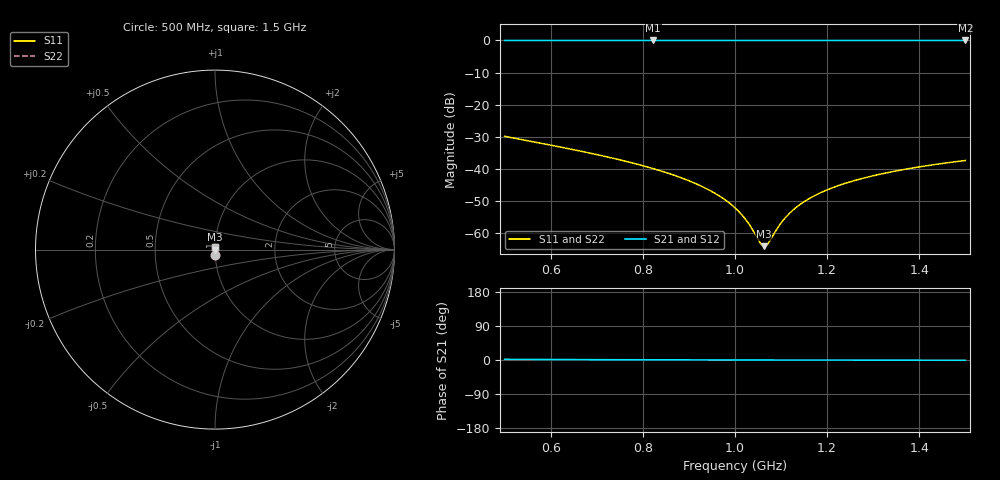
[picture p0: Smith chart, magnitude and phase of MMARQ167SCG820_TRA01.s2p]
! MMARQ167SCG820_TRA01  S-PARAMETER MODEL  ( General Type )
! Model Generated by TAIYO YUDEN Corporation (http://www.ty-top.com)
! Version 1.0
! TAIYO YUDEN Control No. 150609
! Copyright(c) 2015 TAIYO YUDEN CO.,LTD. All Rights Reserved.
! Product Description (link to TY-COMPAS)
! https://ds.yuden.co.jp/TYCOMPAS/or/detail?pn=MMARQ167SCG820JTRA01&u=M
! Products Name : Multilayer Ceramic Capacitors
! Characteristics :
!  Capacitance : 82 pF , Rated Voltage : 250V , TCC : CG / C0G
!  Case Size : 1.6 x 0.8 / 0.063 x 0.031 [mm/inch] , Thickness : 0.7 / 0.028 [mm/inch]
!  (Conditions: Temperature = 25 degC , DC Bias Current/Voltage = 0A / 0V)
! External Node Assignments :
!  1  o---| |---o  2
! GND o---------o GND
! Frequency Range : 500MHz  -  1.5GHz  [ 401 STEP ]
# MHz S RI R 50
! Freq[MHz].  S11 Real  S11 Imag  S21 Real  S21 Imag  S12 Real  S12 Imag  S22 Real  S22 Imag
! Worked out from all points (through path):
!   401 points, 500 MHz to 1.5 GHz, reference 50 ohm
!   highest |S21| = 0.00 dB at 822.5 MHz (marker M1); lowest = 0.0 dB at 1.5 GHz (marker M2)
!   lowest |S11| = -64.1 dB at 1.062 GHz (marker M3), VSWR 1.00, Z = 50.1 - j0.00553 ohm
!   |S11| at or under -10 dB: start of sweep to end of sweep
!   |S22| runs from -64.1 to -29.9 dB; largest |S21 - S12| = 0
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500  0.00139 -0.032  0.9986 0.032  0.9986 0.032  0.00139 -0.032
667.5  0.000768 -0.0187  0.9992 0.0187  0.9992 0.0187  0.000768 -0.0187
822.5  0.000588 -0.01  0.9994 0.01  0.9994 0.01  0.000588 -0.01
835  0.000583 -0.00945  0.9994 0.00945  0.9994 0.00945  0.000583 -0.00945
890  0.00057 -0.00693  0.9994 0.00693  0.9994 0.00693  0.00057 -0.00693
935  0.000571 -0.005  0.9994 0.005  0.9994 0.005  0.000571 -0.005
970  0.000579 -0.00357  0.9994 0.00357  0.9994 0.00357  0.000579 -0.00357
1000  0.000589 -0.00239  0.9994 0.00239  0.9994 0.00239  0.000589 -0.00239
1022.5  0.000599 -0.00154  0.9994 0.00154  0.9994 0.00154  0.000599 -0.00154
1035  0.000605 -0.00107  0.9994 0.00107  0.9994 0.00107  0.000605 -0.00107
1055  0.000616 -0.000328  0.9994 0.000328  0.9994 0.000328  0.000616 -0.000328
1062.5  0.000621 -5.53e-05  0.9994 5.53e-05  0.9994 5.53e-05  0.000621 -5.53e-05
1067.5  0.000624 0.000126  0.9994 -0.000126  0.9994 -0.000126  0.000624 0.000126
1072.5  0.000627 0.000306  0.9994 -0.000306  0.9994 -0.000306  0.000627 0.000306
1097.5  0.000644 0.00119  0.9994 -0.00119  0.9994 -0.00119  0.000644 0.00119
1117.5  0.000659 0.00189  0.9993 -0.00189  0.9993 -0.00189  0.000659 0.00189
1140  0.000677 0.00266  0.9993 -0.00266  0.9993 -0.00266  0.000677 0.00266
1167.5  0.000701 0.00358  0.9993 -0.00358  0.9993 -0.00358  0.000701 0.00358
1200  0.000731 0.00464  0.9993 -0.00464  0.9993 -0.00464  0.000731 0.00464
1237.5  0.000769 0.00583  0.9992 -0.00583  0.9992 -0.00583  0.000769 0.00583
1335  0.000881 0.0088  0.9991 -0.0088  0.9991 -0.0088  0.000881 0.0088
1500  0.00111 0.0134  0.9989 -0.0134  0.9989 -0.0134  0.00111 0.0134
